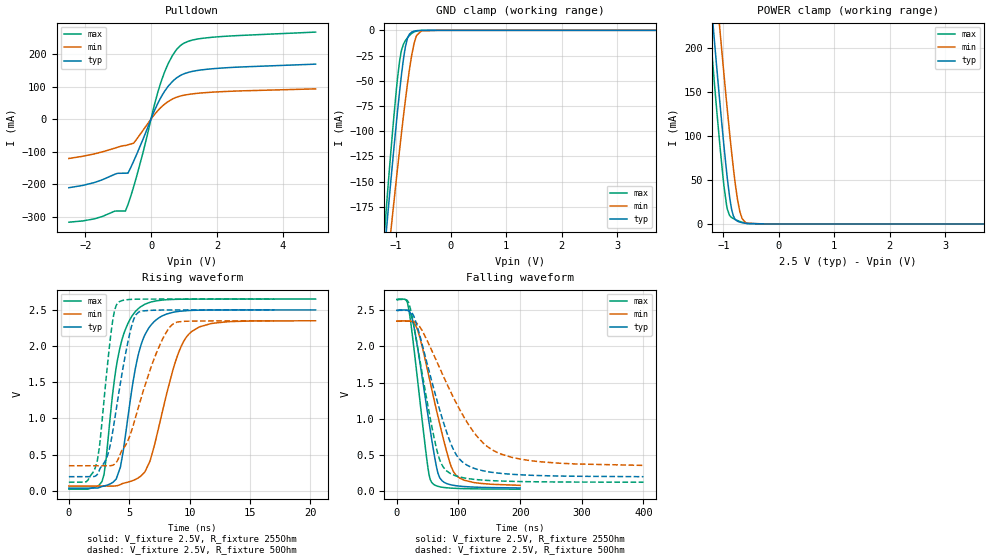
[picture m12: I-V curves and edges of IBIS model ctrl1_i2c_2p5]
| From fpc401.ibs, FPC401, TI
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|   ctrl1_i2c_2p5 Model
[Model]   ctrl1_i2c_2p5
Model_type   I/O_open_drain
Polarity   Non-Inverting
Vinl = 0.54
Vinh = 1.26
Vmeas = 1.25
Vref = 2.5
Cref = 550pF
Rref = 255
|   typ   min   max
|   (nom PVT)   (fast PVT)   (slow PVT)
C_comp   3.353e-12   3.122e-12   3.478e-12
| Where nom  PVT is Nominal Process, 2.5V, 27C
|   Fast PVT is Strong Process,  2.65V, -40C
|   Slow PVT is Weak Process,   2.35V, 125C
[Voltage Range]   2.5   2.35   2.65
|Junction Temperature
[Temperature Range]   27   125   -40
[Pullup Reference]   2.5   2.35   2.65
[Pulldown Reference]   0   0   0
[Power Clamp Reference]   2.5   2.35   2.65
[GND Clamp Reference]   0   0   0
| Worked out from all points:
|   slope of the pulldown table from 0 to 0.375 V, typ, clamps not added: 4.74 ohm
|   GND clamp passes 1 mA (typ) near -0.67 V on its own axis
|   POWER clamp passes 1 mA (typ) near -0.63 V on its own axis
|   falling waveform, V_fixture 2.5V, R_fixture 255Ohm: 20-80 % time 26.9ns typ, 37.3ns min, 21.4ns max; typ from 2.5 V to 0.041 V
|   rising waveform, V_fixture 2.5V, R_fixture 255Ohm: 20-80 % time 1.48ns typ, 2.14ns min, 1.31ns max; typ from 0.037 V to 2.5 V
|   falling waveform, V_fixture 2.5V, R_fixture 50Ohm: 20-80 % time 46.7ns typ, 74.1ns min, 32.6ns max; typ from 2.5 V to 0.197 V
|   rising waveform, V_fixture 2.5V, R_fixture 50Ohm: 20-80 % time 1.41ns typ, 2.34ns min, 920ps max; typ from 0.196 V to 2.5 V
[Pulldown]
|   Voltage   I(typ)   I(min)   I(max)
-2.5V     -211.1mA   -121.3mA   -317.2mA
-780mV    -166.5mA   -81.39mA   -282.8mA
-703.3mV  -166.4mA   -79.19mA   -262.8mA
-530.7mV  -129.5mA   -74.24mA   -208.2mA
-247.5mV  -62.48mA   -34.79mA   -103.6mA
100mV     25.49mA    13.64mA    43.63mA
292.5mV   65.56mA    35.16mA    111.4mA
535mV     102.8mA    55mA       173.8mA
892mV     134.3mA    70.91mA    226.2mA
1.248V    146.6mA    77.39mA    242.8mA
1.847V    154.7mA    82.69mA    251.6mA
5V        169mA      92.88mA    267.6mA
[GND Clamp]
|   Voltage   I(typ)   I(min)   I(max)
-2.5V     -1.076A    -999.1mA   -1.173A
-1.4V     -346.1mA   -370.4mA   -343mA
-1.133V   -178.4mA   -224.7mA   -152.9mA
-1.097V   -157mA     -205.9mA   -129mA
-1.052V   -130.5mA   -182.5mA   -99.78mA
-985mV    -91.97mA   -147.8mA   -58.97mA
-923.2mV  -58.98mA   -116.9mA   -29.3mA
-819.9mV  -15.92mA   -68.35mA   -10.12mA
-705.9mV  -1.65mA    -24.05mA   -3.017mA
-627.5mV  -378.3uA   -6.231mA   -803.9uA
-530.7mV  -48.81uA   -526.9uA   -88.92uA
5V        0A         0A         0A
[POWER Clamp]
|   Voltage   I(typ)   I(min)   I(max)
-2.5V     1.257A     1.315A     1.24A
-1.4V     385.6mA    465.7mA    341.5mA
-1.159V   205.3mA    288.3mA    156.9mA
-1.062V   136.2mA    219.1mA    87.67mA
-987.5mV  86.55mA    167.9mA    41.5mA
-928.5mV  51.09mA    128.7mA    16.6mA
-845.6mV  14.85mA    77.42mA    7.025mA
-793.9mV  5.674mA    49.25mA    5.223mA
-745.7mV  3.042mA    27.55mA    3.847mA
-662.3mV  1.416mA    6.079mA    1.934mA
-563.6mV  434.9uA    773.4uA    531.7uA
5V        0A         0A         0A
[Ramp]
R_load = 255
|   typ   min   max
dV/dt_r   1.47754/1.47687e-09   1.37049/2.13875e-09   1.57614/1.3127e-09
dV/dt_f   1.47513/2.68481e-08   1.36344/3.73295e-08   1.5752/2.13582e-08
[Falling Waveform]
V_fixture = 2.5V
V_fixture_min = 2.35V
V_fixture_max = 2.65V
R_fixture = 255Ohm
|   Time   V(typ)   V(min)   V(max)
0s        2.5V       2.35V      2.65V
15.14ns   2.504V     2.354V     2.644V
19.88ns   2.49V      2.353V     2.501V
33.65ns   1.988V     2.232V     1.54V
50.08ns   1.072V     1.664V     348mV
56.6ns    715mV      1.411V     117.7mV
69.78ns   179.6mV    921.9mV    57.4mV
85.26ns   90.13mV    413.5mV    40.88mV
95.78ns   72.68mV    220.7mV    35.82mV
200ns     41.45mV    77.61mV    24.67mV
[Rising Waveform]
V_fixture = 2.5V
V_fixture_min = 2.35V
V_fixture_max = 2.65V
R_fixture = 255Ohm
|   Time   V(typ)   V(min)   V(max)
0s        37.44mV    65.85mV    23.1mV
2.744ns   60.1mV     65.91mV    129.6mV
3.088ns   75.1mV     65.92mV    447.7mV
3.915ns   162.3mV    68.65mV    1.702V
4.664ns   742.2mV    110.3mV    2.223V
5.883ns   1.966V     195mV      2.535V
7.314ns   2.375V     789.7mV    2.628V
8.816ns   2.473V     1.782V     2.646V
10.16ns   2.493V     2.201V     2.649V
20.42ns   2.5V       2.35V      2.65V
[Falling Waveform]
V_fixture = 2.5V
V_fixture_min = 2.35V
V_fixture_max = 2.65V
R_fixture = 50Ohm
|   Time   V(typ)   V(min)   V(max)
0s        2.5V       2.35V      2.65V
16.75ns   2.5V       2.351V     2.64V
22.05ns   2.488V     2.35V      2.525V
35.98ns   2.193V     2.292V     1.885V
63.23ns   1.314V     1.822V     628.1mV
80.22ns   829.4mV    1.501V     281.9mV
105.5ns   407.9mV    1.075V     187.1mV
132ns     295.8mV    737.1mV    155.2mV
162.5ns   248.8mV    533.9mV    139.4mV
400ns     197.3mV    353.6mV    120.9mV
[Rising Waveform]
V_fixture = 2.5V
V_fixture_min = 2.35V
V_fixture_max = 2.65V
R_fixture = 50Ohm
|   Time   V(typ)   V(min)   V(max)
0s        195.6mV    346.7mV    120.3mV
1.454ns   195.6mV    346.7mV    127mV
2.229ns   207.7mV    346.7mV    339.5mV
2.529ns   286.8mV    346.7mV    602.9mV
3.593ns   783.5mV    352.3mV    2.31V
4.132ns   1.35V      456mV      2.608V
5.562ns   2.436V     1.04V      2.648V
7.268ns   2.497V     1.914V     2.65V
8.596ns   2.499V     2.302V     2.65V
17.02ns   2.5V       2.35V      2.65V
